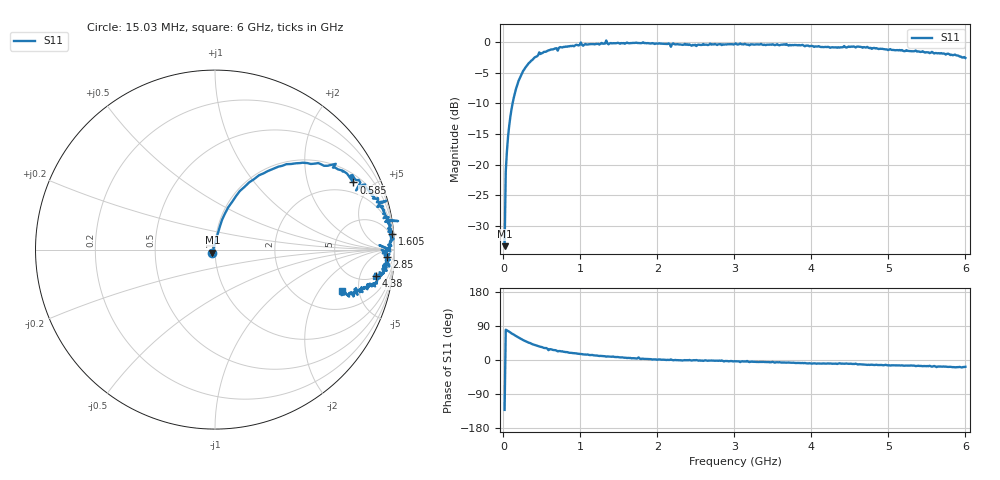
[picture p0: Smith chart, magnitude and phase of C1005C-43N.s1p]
!	Network	Analyzer	HP8753E.07.74:	Oct	30	2002	Serial	No.	JP38451487
!	Hewlett-Packard
!	7	Sep	2009	9:08:14
!	Frequency	S11
#	HZ	S	RI	R	50
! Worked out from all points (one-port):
!   400 points, 15.03 MHz to 6 GHz, reference 50 ohm
!   lowest |S11| = -33.3 dB at 15.03 MHz (marker M1), VSWR 1.04, Z = 48.6 - j1.57 ohm
!   |S11| at or under -10 dB: start of sweep to 118.5 MHz
!   S11 on the Smith chart (normalised r, x): 15.03 MHz: 0.97, -0.03; 585 MHz: 1.38, +3.89; 1.605 GHz: 2, +22; 2.85 GHz: 23, -24; 4.38 GHz: 5, -9; 6 GHz: 3.25, -3.31
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1.502992e7  -0.0144 -0.0162
3.002985e7  0.0154 0.0867
4.502978e7  0.0263 0.126
9.002955e7  0.074 0.236
1.350293e8  0.138 0.326
3.150284e8  0.452 0.481
4.650277e8  0.673 0.478
5.850271e8  0.771 0.374
7.650262e8  0.834 0.352
1.005025e9  0.956 0.272
1.035025e9  0.904 0.238
1.320023e9  0.96 0.166
1.335023e9  1.02 0.159
1.365023e9  0.948 0.155
1.515022e9  0.964 0.117
1.605022e9  0.988 0.0886
1.755021e9  0.976 0.118
1.785021e9  0.98 0.0464
2.145019e9  0.976 0.00317
2.175019e9  0.916 0.0247
2.265019e9  0.963 -0.00681
2.850016e9  0.959 -0.0424
3.015015e9  0.975 -0.0567
3.765011e9  0.937 -0.116
4.380008e9  0.896 -0.148
4.515007e9  0.907 -0.156
5.265004e9  0.819 -0.215
6e9  0.707 -0.228
